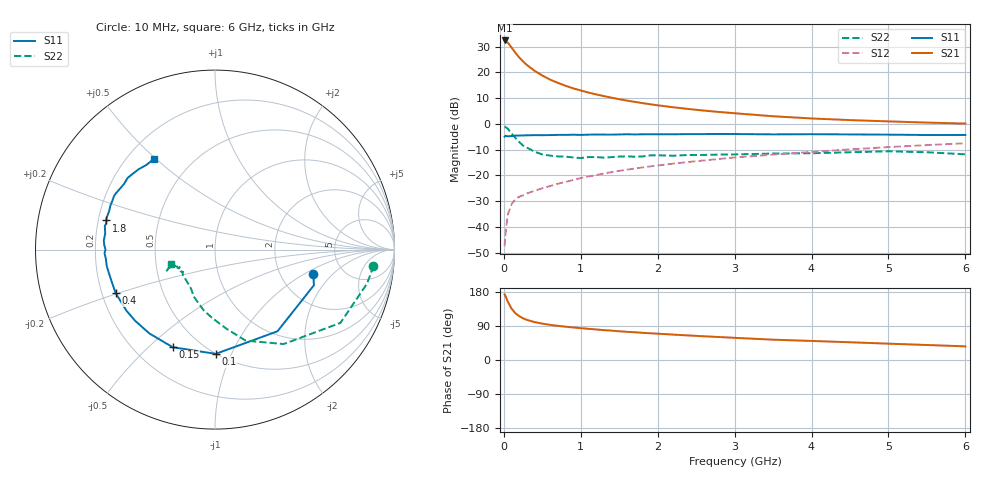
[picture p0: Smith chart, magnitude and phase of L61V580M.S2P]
!  INFINEON TECHNOLOGIES Small Signal Semiconductors
! BFR380L3 , Si-NPN RF-Transistor in TSLP-3-1
!  Vce=1.5 V,  Ic=80 mA
! Common Emitter S-Parameters:  07. March 2005
#  GHz  S  MA  R  50
! f  S11  S21  S12  S22
! GHz  Mag  Ang  Mag  Ang  Mag  Ang  Mag  Ang
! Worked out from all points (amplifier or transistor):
!   36 points, 10 MHz to 6 GHz, reference 50 ohm
!   highest |S21| = 32.4 dB at 10 MHz (marker M1)
!   |S21| within 3 dB of that: start of sweep to 106.4 MHz
!   unconditionally stable (mu >= 1): 982.3 MHz to 5.956 GHz
!   at 250 MHz: K = 0.55, MSG = 26.0 dB, |S12| = -27.8 dB
!   at 1.4 GHz: K = 1.05, MAG = 13.1 dB, |S12| = -18.8 dB
!   at 6 GHz: K = 1.00, MSG = 3.8 dB, |S12| = -7.5 dB
!   S11 on the Smith chart (normalised r, x): 10 MHz: 3.05, -1.22; 100 MHz: 0.50, -0.87; 150 MHz: 0.36, -0.60; 400 MHz: 0.26, -0.20; 1.8 GHz: 0.23, +0.12; 6 GHz: 0.31, +0.49
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0.01  0.5643 -14.0  41.79 173.1  0.0042 64.5  0.8875 -5.8
0.02  0.5858 -19.8  41.51 169.6  0.0068 77.3  0.8687 -12.5
0.05  0.573 -52.6  38.04 154.3  0.0169 66.2  0.8094 -30.3
0.1  0.5809 -89.6  30.48 135.6  0.0274 56.0  0.6505 -54.0
0.15  0.5926 -113.4  24.12 123.4  0.0344 51.1  0.5351 -71.4
0.2  0.5931 -127.9  19.55 115.6  0.0383 48.4  0.4445 -81.9
0.25  0.5963 -138.4  16.36 110.0  0.0409 47.7  0.3784 -92.9
0.3  0.5993 -145.5  13.9 105.9  0.0444 48.6  0.3456 -100.3
0.4  0.6042 -156.3  10.74 100.0  0.0501 50.3  0.2877 -114.2
0.5  0.6028 -163.1  8.704 96.0  0.056 53.1  0.2545 -121.7
0.6  0.6058 -168.0  7.265 92.8  0.0617 55.3  0.2414 -128.3
0.7  0.6102 -171.2  6.281 90.2  0.0684 57.7  0.233 -134.9
0.9  0.6159 -178.2  4.909 85.9  0.0807 60.7  0.2223 -144.3
1.1  0.6176 177.6  4.06 82.2  0.0946 62.4  0.2264 -147.5
1.4  0.6179 171.9  3.224 77.6  0.115 64.1  0.2257 -152.3
1.8  0.6268 165.0  2.536 71.8  0.1424 65.1  0.2323 -156.8
2.2  0.6278 159.7  2.105 67.0  0.1686 65.1  0.2404 -157.4
2.8  0.6369 152.1  1.703 60.6  0.208 64.9  0.2528 -160.6
3.5  0.6249 144.1  1.406 53.6  0.2526 62.6  0.2648 -158.7
4.5  0.6237 137.6  1.184 46.8  0.3194 60.4  0.2805 -157.5
5.5  0.6074 129.1  1.059 39.6  0.3863 56.1  0.2807 -157.9
6  0.6087 124.0  1.014 36.0  0.4201 53.7  0.2562 -162.1
